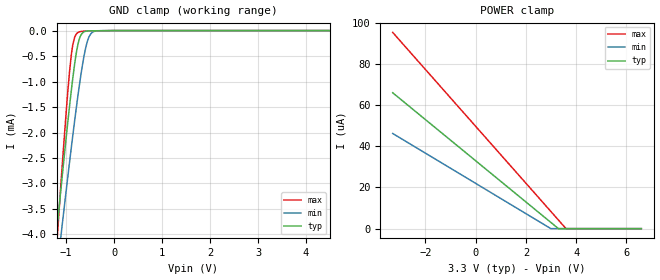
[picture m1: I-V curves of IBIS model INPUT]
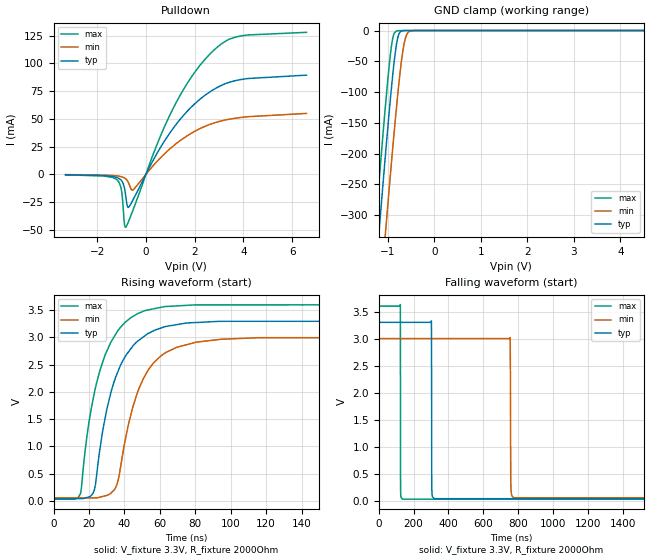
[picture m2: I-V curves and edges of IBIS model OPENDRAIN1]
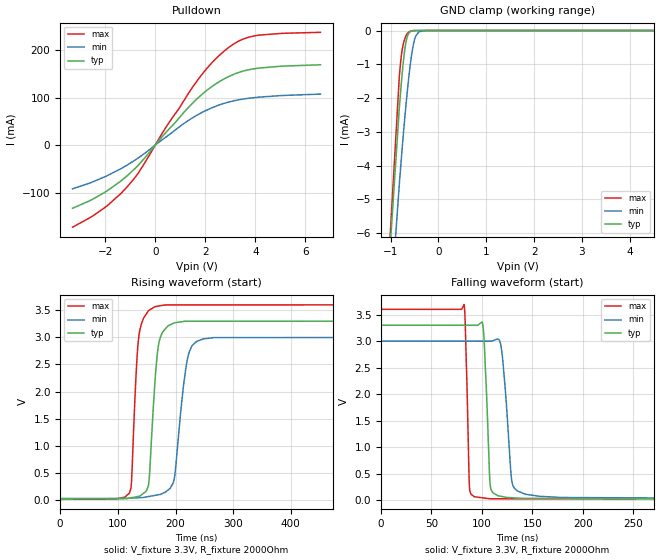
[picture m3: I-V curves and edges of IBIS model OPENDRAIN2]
|Texas Instruments Incorporated
|DRV8313 2.5-A Triple 1/2-H Bridge Driver
[IBIS Ver]   4.1
[File name]   drv8313.ibs
[Date]   09/07/2018
[File Rev]   1.0
[Source]
| Texas Instruments Incorporated.
| Analog-eLab Design Center, HPA
| 12500 TI Blvd
| Dallas, TX -75243
[Notes]   Revision History:
| Rev 1.0: 09/07/2018
| - Initial version of the model
| - Model generated from simulations in SPECTRE
| - C_comp although listed in numerical order of value are
|   obtained from varying PVT conditions. For PVT conditions for
|   each specific value refer the buffer description under
|   respective [Model]. IBIS model user is responsible for using
|   appropriate C_comp to simulate for Signal Integrity.
| - Warnings regarding combined Non-monotonicity of various models
|   have been reviewed and considered minor and can be ignored.
[Disclaimer]
| This model is designed as an aid for customers of Texas Instruments.
| TI and its licensors and suppliers make no warranties, either expressed
| or implied, with respect to this  model, including the warranties of
| merchantability or fitness for a particular purpose. The model is
| provided solely on an "as is" basis. The entire risk as to its quality
| and performance is with the customer.
| This model is subject to change without notice. Texas Instruments
| Incorporated is not responsible for updating this model.
[Copyright]
(C) Copyright 2018 Texas Instruments Incorporated.All rights reserved.
|  Component DRV8313PWPR 28-pin HTSSOP - PWP package
|  Part # DRV8313PWPR
[Component]   DRV8313PWPR
[Manufacturer]  TI
[Package]   |28-pin HTSSOP - PWP package
|   typ   min   max
R_pkg   0.05   0.04   0.06
L_pkg   1.0nH   0.8nH   1.2nH
C_pkg   0.2pF   0.16pF   0.24pF
[Pin] signal_name  model_name   R_pin   L_pin   C_pin
1   CPL   POWER   NA   NA   NA
2   CPH   POWER   NA   NA   NA
3   VCP   POWER   NA   NA   NA
4   VM   POWER   NA   NA   NA
5   OUT1   NC   NA   NA   NA
6   PGND1   GND   NA   NA   NA
7   PGND2   GND   NA   NA   NA
8   OUT2   NC   NA   NA   NA
9   OUT3   NC   NA   NA   NA
10   PGND3   GND   NA   NA   NA
11   VM   POWER   NA   NA   NA
12   COMPP   NC   NA   NA   NA
13   COMPN   NC   NA   NA   NA
14   GND   GND   NA   NA   NA
15   V3P3   POWER   NA   NA   NA
16   nRESET   INPUT   NA   NA   NA
17   nSLEEP   INPUT   NA   NA   NA
18   nFAULT   OPENDRAIN1   NA   NA   NA
19   nCOMPO   OPENDRAIN2   NA   NA   NA
20   GND   GND   NA   NA   NA
21   NC   NC   NA   NA   NA
22   EN3   INPUT   NA   NA   NA
23   IN3   INPUT   NA   NA   NA
24   EN2   INPUT   NA   NA   NA
25   IN2   INPUT   NA   NA   NA
26   EN1   INPUT   NA   NA   NA
27   IN1   INPUT   NA   NA   NA
28   GND   GND   NA   NA   NA
|  Component DRV8313RHHR 36-pin VQFN - RHH package
|  Part # DRV8313RHHR
[Component]   DRV8313RHHR
[Manufacturer]  TI
[Package]   |36-pin VQFN - RHH package
|   typ   min   max
R_pkg   0.05   0.04   0.06
L_pkg   1.0nH   0.8nH   1.2nH
C_pkg   0.2pF   0.16pF   0.24pF
[Pin] signal_name  model_name   R_pin   L_pin   C_pin
1   EN1   INPUT   NA   NA   NA
2   IN1   INPUT   NA   NA   NA
3   GND   GND   NA   NA   NA
4   NC   NC   NA   NA   NA
5   CPL   POWER   NA   NA   NA
6   CPH   POWER   NA   NA   NA
7   VCP   POWER   NA   NA   NA
8   NC   NC   NA   NA   NA
9   VM   POWER   NA   NA   NA
10   OUT1   NC   NA   NA   NA
11   PGND1   POWER   NA   NA   NA
12   PGND2   POWER   NA   NA   NA
13   OUT2   NC   NA   NA   NA
14   NC   NC   NA   NA   NA
15   OUT3   NC   NA   NA   NA
16   PGND3   POWER   NA   NA   NA
17   GND   POWER   NA   NA   NA
18   RSVD   NC   NA   NA   NA
19   VM   POWER   NA   NA   NA
20   GND   POWER   NA   NA   NA
21   COMPP   NC   NA   NA   NA
22   COMPN   NC   NA   NA   NA
23   GND   POWER   NA   NA   NA
24   GND   POWER   NA   NA   NA
25   V3P3   POWER   NA   NA   NA
26   nRESET   INPUT   NA   NA   NA
27   nSLEEP   INPUT   NA   NA   NA
28   nFAULT   OPENDRAIN1   NA   NA   NA
29   nCOMPO   OPENDRAIN2   NA   NA   NA
30   GND   POWER   NA   NA   NA
31   GND   POWER   NA   NA   NA
32   GND   POWER   NA   NA   NA
33   EN3   INPUT   NA   NA   NA
34   IN3   INPUT   NA   NA   NA
35   EN2   INPUT   NA   NA   NA
36   IN2   INPUT   NA   NA   NA
| Models and submodels in the file (3): INPUT (Input), OPENDRAIN1 (Open_drain), OPENDRAIN2 (Open_drain)
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|   in1 Model
[Model]   INPUT
Model_type   Input
Vinl = 0.7
Vinh = 2.2
|   typ   min   max
C_comp   2.268pF   2.040pF   2.499pF
|  Where Nom  PVT is Nominal Process, 3.3,  27C
|   Fast PVT is Strong Process,  3.6, -40C
|   Slow PVT is Weak Process,   3V, 125C
[Model spec]
|subparameter
Vinl   0.7   0.64   0.76
Vinh   2.2   2.0   2.4
[Voltage Range]   3.3   3   3.6
|Junction Temperature
[Temperature Range]   27   125   -40
[Power Clamp Reference]   3.3   3   3.6
[GND Clamp Reference]   0   0   0
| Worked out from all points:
|   GND clamp passes 1 mA (typ) near -0.87 V on its own axis
[GND Clamp]
|   Voltage   I(typ)   I(min)   I(max)
-3.3V     -25.59mA   -23.01mA   -35.32mA
-1.27V    -4.675mA   -5.388mA   -5.244mA
-1.112V   -3.146mA   -4.065mA   -3.056mA
-1.092V   -2.959mA   -3.902mA   -2.792mA
-973.5mV  -1.871mA   -2.938mA   -1.296mA
-894.3mV  -1.196mA   -2.315mA   -499uA
-825mV    -673.7uA   -1.789mA   -138.6uA
-735.9mV  -202.3uA   -1.156mA   -29.36uA
-636.9mV  -30.32uA   -552.1uA   -11.78uA
-557.7mV  -8.639uA   -214.3uA   -8.123uA
-399.3mV  -3.961uA   -12.59uA   -5.445uA
6.59V     0A         0A         0A
[POWER Clamp]
|   Voltage   I(typ)   I(min)   I(max)
-3.3V     66uA       46.25uA    95.3uA
2.986V    3.08uA     31.47nA    8.425uA
3.293V    3.52nA     0A         4.182uA
3.59V     0A         0A         74.24nA
6.59V     0A         0A         0A
|   OPENDRAIN1 Model
[Model]   OPENDRAIN1
Model_type   Open_drain
Polarity   Inverting
Vmeas = 1.65
Vref = 3.3
Cref = 15pF
Rref = 2000
|   typ   min   max
C_comp   2.386pF   2.058pF   2.739pF
|  Where Nom  PVT is Nominal Process, 3.3,  27C
|   Fast PVT is Strong Process,  3.6, -40C
|   Slow PVT is Weak Process,   3V, 125C
[Voltage Range]   3.3   3   3.6
|Junction Temperature
[Temperature Range]   27   125   -40
[Pullup Reference]   3.3   3   3.6
[Pulldown Reference]   0   0   0
[Power Clamp Reference]   3.3   3   3.6
[GND Clamp Reference]   0   0   0
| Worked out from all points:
|   slope of the pulldown table from 0 to 0.495 V, typ, clamps not added: 24.3 ohm
|   GND clamp passes 1 mA (typ) near -0.71 V on its own axis
|   falling waveform, V_fixture 3.3V, R_fixture 2000Ohm: 20-80 % time 1.03ns typ, 1.76ns min, 684ps max; typ from 3.3 V to 0.037 V
|   rising waveform, V_fixture 3.3V, R_fixture 2000Ohm: 20-80 % time 15.3ns typ, 15.7ns min, 14.8ns max; typ from 0.037 V to 3.3 V
[Pulldown]
|   Voltage   I(typ)   I(min)   I(max)
-3.3V     -429.4uA   -298uA     -519.9uA
-1.191V   -2.915mA   -1.463mA   -4.851mA
-1.013V   -5.455mA   -2.168mA   -13.46mA
-884.4mV  -12.23mA   -3.265mA   -44.45mA
-825mV    -20.35mA   -4.191mA   -47.63mA
-735.9mV  -29.81mA   -6.777mA   -43.58mA
-528mV    -22.85mA   -14.04mA   -32.02mA
976.8mV   37.07mA    22.79mA    53.13mA
1.7V      56.86mA    34.78mA    82.05mA
2.501V    72.39mA    43.88mA    105.4mA
3.749V    84.72mA    50.74mA    123.9mA
6.59V     89.29mA    54.83mA    127.9mA
[GND Clamp]
|   Voltage   I(typ)   I(min)   I(max)
-3.3V     -2.384A    -2.505A    -2.308A
-1.379V   -503.3mA   -631.6mA   -421.9mA
-1.231V   -363.3mA   -491.7mA   -281.6mA
-1.211V   -344.8mA   -473.2mA   -263.1mA
-1.171V   -308.2mA   -436.4mA   -226.6mA
-1.063V   -209.3mA   -336.5mA   -129.1mA
-924mV    -92.08mA   -213.5mA   -24.63mA
-825mV    -26.11mA   -131.3mA   -1.164mA
-755.7mV  -4.41mA    -79.36mA   -292.2uA
-656.7mV  -167.7uA   -23.13mA   -52.28uA
-508.2mV  -1.87uA    -659.7uA   -806.5nA
6.59V     0A         0A         0A
[POWER Clamp]
|   Voltage   I(typ)   I(min)   I(max)
-3.3V     0A         0A         0A
0V        0A         0A         0A
6.59V     0A         0A         0A
[Ramp]
R_load = 2000
|   typ   min   max
dV/dt_r   1.95799/1.53364e-08   1.76769/1.57397e-08   2.14309/1.47548e-08
dV/dt_f   1.95799/1.02529e-09   1.76769/1.75703e-09   2.14309/6.81479e-10
[Falling Waveform]
V_fixture = 3.3V
V_fixture_min = 3V
V_fixture_max = 3.6V
R_fixture = 2000Ohm
C_fixture = 0F
|   Time   V(typ)   V(min)   V(max)
0s        3.3V       3V         3.6V
124ns     3.3V       3V         3.63V
125.9ns   3.3V       3V         187mV
136.3ns   3.3V       3V         30.87mV
302.3ns   3.324V     3V         30.78mV
305.1ns   210.4mV    3V         30.78mV
318.3ns   39.92mV    3V         30.77mV
754ns     39.62mV    3.019V     30.53mV
777.3ns   39.6mV     57.29mV    30.52mV
5us       36.69mV    53.85mV    28.18mV
[Rising Waveform]
V_fixture = 3.3V
V_fixture_min = 3V
V_fixture_max = 3.6V
R_fixture = 2000Ohm
C_fixture = 0F
|   Time   V(typ)   V(min)   V(max)
0s        36.69mV    53.85mV    28.18mV
15.01ns   39.74mV    54.35mV    119.2mV
22.43ns   150.5mV    54.6mV     1.879V
30.15ns   1.691V     100.2mV    2.75V
35.9ns    2.336V     312.6mV    3.102V
42.51ns   2.742V     1.438V     3.33V
50.59ns   3.003V     2.235V     3.475V
62.17ns   3.186V     2.695V     3.559V
79.81ns   3.268V     2.903V     3.593V
2us       3.3V       3V         3.6V
|   OPENDRAIN2 Model
[Model]   OPENDRAIN2
Model_type   Open_drain
Polarity   Inverting
Vmeas = 1.65
Vref = 3.3
Cref = 2pF
Rref = 2000
|   typ   min   max
C_comp   0.124pF   0.106pF   0.187pF
| Where Nom  PVT is Nominal Process, 3.3V,  27C
|   Fast PVT is Strong Process,  3.0V, -40C
|   Slow PVT is Weak Process,   3.6V, 125C
[Voltage Range]   3.3   3   3.6
|Junction Temperature
[Temperature Range]   27   125   -40
[Pullup Reference]   3.3   3   3.6
[Pulldown Reference]   0   0   0
[Power Clamp Reference]   3.3   3   3.6
[GND Clamp Reference]   0   0   0
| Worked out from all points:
|   slope of the pulldown table from 0 to 0.495 V, typ, clamps not added: 16.2 ohm
|   GND clamp passes 1 mA (typ) near -0.74 V on its own axis
|   falling waveform, V_fixture 3.3V, R_fixture 2000Ohm: 20-80 % time 4.09ns typ, 6.59ns min, 2.79ns max; typ from 3.3 V to 0.024 V
|   rising waveform, V_fixture 3.3V, R_fixture 2000Ohm: 20-80 % time 12ns typ, 17.2ns min, 9.79ns max; typ from 0.024 V to 3.3 V
[Pulldown]
|   Voltage   I(typ)   I(min)   I(max)
-3.3V     -133.2mA   -92.29mA   -173.1mA
-2.509V   -114.5mA   -77.91mA   -150mA
-1.984V   -98.72mA   -66.17mA   -130.8mA
-1.103V   -63.95mA   -41.56mA   -87.07mA
-677.5mV  -42.56mA   -27.01mA   -59.05mA
431.3mV   26.96mA    17.13mA    37.76mA
1.679V    98.23mA    63.54mA    136.1mA
2.233V    122.5mA    78.09mA    172mA
2.906V    144mA      90.51mA    205mA
3.471V    155.7mA    96.91mA    223mA
4.035V    161.9mA    100.7mA    231.3mA
6.599V    169.6mA    107.7mA    238.1mA
[GND Clamp]
|   Voltage   I(typ)   I(min)   I(max)
-3.3V     -87.96mA   -75mA      -105.8mA
-1.014V   -6.508mA   -8.449mA   -6.199mA
-816.1mV  -2.259mA   -4.521mA   -1.328mA
-786.4mV  -1.734mA   -3.985mA   -878.1uA
-746.8mV  -1.111mA   -3.299mA   -485.2uA
-687.4mV  -416.4uA   -2.341mA   -185.5uA
-647.8mV  -165.9uA   -1.761mA   -84.31uA
-588.4mV  -31.98uA   -1.007mA   -19.53uA
-538.9mV  -7.314uA   -526.5uA   -4.659uA
-469.6mV  -883.3nA   -150.9uA   -444.4nA
-261.7mV  0A         -826nA     0A
6.599V    0A         0A         0A
[POWER Clamp]
|   Voltage   I(typ)   I(min)   I(max)
-3.3V     0A         0A         0A
0V        0A         0A         0A
6.59V     0A         0A         0A
[Ramp]
R_load = 2000
|   typ   min   max
dV/dt_r   1.96535/1.19261e-08   1.77905/1.70864e-08   2.14853/9.75146e-09
dV/dt_f   1.96535/4.07963e-09   1.77905/6.59293e-09   2.14853/2.7859e-09
[Falling Waveform]
V_fixture = 3.3V
V_fixture_min = 3V
V_fixture_max = 3.6V
R_fixture = 2000Ohm
C_fixture = 0F
|   Time   V(typ)   V(min)   V(max)
0s        3.3V       3V         3.6V
82.28ns   3.299V     2.999V     3.691V
83.53ns   3.299V     2.999V     3.306V
87.94ns   3.299V     2.999V     196.8mV
101.1ns   3.287V     2.999V     46.53mV
107.8ns   400.6mV    2.999V     29.8mV
118.7ns   75.85mV    2.939V     29.77mV
130.9ns   47.53mV    268.4mV    29.75mV
178.9ns   34.33mV    53.94mV    29.64mV
5us       24.42mV    34.92mV    19.11mV
[Rising Waveform]
V_fixture = 3.3V
V_fixture_min = 3V
V_fixture_max = 3.6V
R_fixture = 2000Ohm
C_fixture = 0F
|   Time   V(typ)   V(min)   V(max)
0s        24.42mV    34.92mV    19.11mV
120.6ns   42.18mV    39.88mV    145.8mV
135.5ns   72.74mV    47.77mV    2.932V
149.6ns   176.4mV    63.87mV    3.429V
168.7ns   2.709V     99.95mV    3.568V
182.2ns   3.149V     150.4mV    3.592V
197.5ns   3.261V     378.6mV    3.592V
223.8ns   3.292V     2.731V     3.592V
267.1ns   3.292V     2.992V     3.592V
5us       3.3V       3V         3.6V
